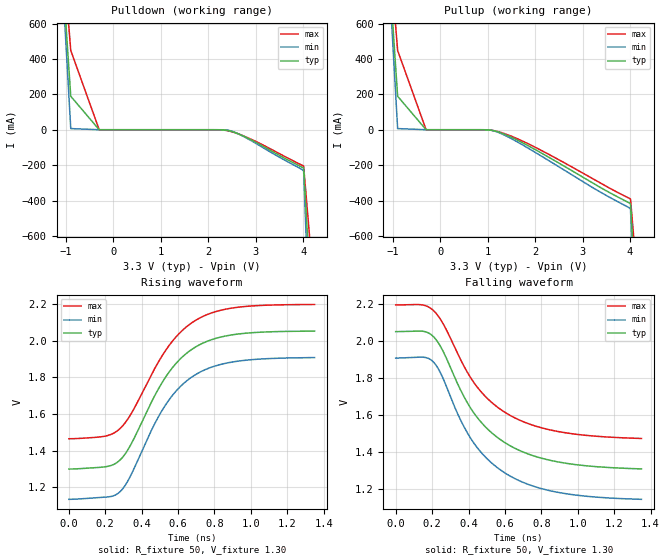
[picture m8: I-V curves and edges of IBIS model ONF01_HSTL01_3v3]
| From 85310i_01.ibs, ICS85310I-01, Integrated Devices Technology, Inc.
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[Model]   ONF01_HSTL01_3v3
Model_type   Output_ECL
Polarity   Non-Inverting
|   typ   min   max
C_comp   2pF   1.5pF   2.5pF
Vmeas = 1.61V
Rref = 50
Cref = 0
Vref = 1.3V
|   typ   min   max
[Voltage range]   3.3V   3.135V   3.465V
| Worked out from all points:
|   rising waveform, R_fixture 50, V_fixture 1.30: 20-80 % time 264ps typ, 264ps min, 270ps max; typ from 1.3 V to 2.05 V
|   falling waveform, R_fixture 50, V_fixture 1.30: 20-80 % time 309ps typ, 306ps min, 312ps max; typ from 2.05 V to 1.31 V
[Pulldown]
|Voltage   I (typ)   I (min)   I (max)
-3.3V     9.786A     12.03A     8.45A
-1.5V     2.58A      2.839A     2.441A
-900mV    189.2mA    6.554mA    448mA
-300mV    38.6nA     139.1pA    1.11uA
2.176V    -32.47uA   -2.906uA   -126.3uA
2.471V    -8.172mA   -6.15mA    -9.576mA
2.669V    -27.44mA   -27.9mA    -26.99mA
2.964V    -65.77mA   -71.18mA   -61.41mA
4.01V     -217mA     -232.2mA   -205.2mA
4.528V    -2.645A    -3.887A    -1.854A
6.6V      -15.69A    -20.55A    -12.72A
[Pullup]
|Voltage   I (typ)   I (min)   I (max)
-3.3V     9.786A     12.03A     8.45A
-1.5V     2.58A      2.839A     2.441A
-900mV    189.2mA    6.554mA    448mA
-300mV    38.6nA     139.1pA    1.11uA
1.041V    -1.702mA   -1.46mA    -1.79mA
1.288V    -18.86mA   -22.48mA   -16.25mA
1.682V    -66.67mA   -77.83mA   -57.91mA
2.274V    -153.5mA   -172.3mA   -137.3mA
3.26V     -308.3mA   -334.7mA   -283.6mA
4.01V     -417.3mA   -447.3mA   -391.2mA
4.528V    -2.844A    -4.101A    -2.041A
6.6V      -15.79A    -20.6A     -12.84A
[Ramp]
|   typ   min   max
dV/dt_r   0.601/0.412n   0.617/0.414n   0.585/0.421n
dV/dt_f   0.598/0.504n   0.617/0.497n   0.581/0.51n
R_load =   50.0000
[Rising Waveform]
R_fixture = 50
V_fixture = 1.30   | VCC_typ - 2V
V_fixture_max = 1.465   | VCC_max - 2V
V_fixture_min = 1.135   | VCC_min - 2V
C_fixture = 0.0p
| Time   typ   min   max
0s        1.3V       1.135V     1.465V
200ps     1.312V     1.146V     1.479V
283.8ps   1.352V     1.179V     1.523V
345.9ps   1.443V     1.277V     1.607V
458.1ps   1.673V     1.52V      1.822V
528.4ps   1.796V     1.645V     1.941V
610.8ps   1.899V     1.748V     2.043V
702.7ps   1.969V     1.818V     2.114V
921.6ps   2.035V     1.887V     2.181V
1.35ns    2.051V     1.907V     2.196V
[Falling Waveform]
R_fixture = 50
V_fixture = 1.30   | VCC_typ - 2V
V_fixture_max = 1.465   | VCC_max - 2V
V_fixture_min = 1.135   | VCC_min - 2V
C_fixture = 0.0p
| Time   typ   min   max
0s        2.052V     1.909V     2.197V
148.6ps   2.054V     1.913V     2.197V
206.8ps   2.025V     1.888V     2.167V
262.2ps   1.942V     1.794V     2.092V
347.3ps   1.754V     1.591V     1.918V
420.3ps   1.624V     1.46V      1.789V
512.2ps   1.516V     1.352V     1.681V
623ps     1.436V     1.271V     1.601V
898.6ps   1.344V     1.178V     1.509V
1.35ns    1.307V     1.142V     1.472V
